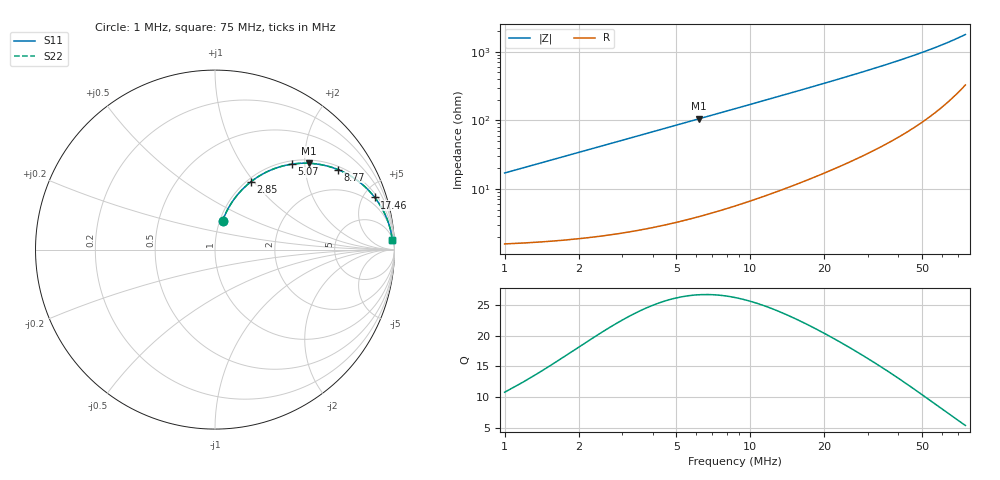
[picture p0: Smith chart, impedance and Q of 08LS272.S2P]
! Coilcraft 0805LS-272 Chip Inductor
! 18 September 2002
# MHZ S MA R 50
!Freq  MagS11  AngS11  MagS21  AngS21  MagS12  AngS12  MagS22  AngS22
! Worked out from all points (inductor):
!   401 points, 1 MHz to 75 MHz, reference 50 ohm
!   read as one part in series: L = 2.7 uH near 1.37 MHz
!   highest Q = 26.7 at 6.18 MHz (marker M1), where L = 2.7 uH
!   S11 on the Smith chart (normalised r, x): 1 MHz: 1.03, +0.34; 2.85 MHz: 1.04, +0.97; 5.07 MHz: 1.07, +1.72; 8.77 MHz: 1.11, +2.99; 17.46 MHz: 1.28, +6.02; 75 MHz: 8, +35
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1  0.1654 75.2  0.971 -9.5  0.971 -9.5  0.1654 75.2
1.185  0.1947 74.2  0.9653 -11.2  0.9653 -11.2  0.1947 74.2
1.555  0.2515 71.7  0.9515 -14.5  0.9515 -14.5  0.2515 71.7
1.925  0.3058 69.0  0.935 -17.8  0.935 -17.8  0.3058 69.0
2.295  0.3572 66.2  0.9161 -20.9  0.9161 -20.9  0.3572 66.2
2.85  0.4281 62.1  0.8845 -25.3  0.8845 -25.3  0.4281 62.1
3.775  0.5301 55.7  0.8266 -32.0  0.8266 -32.0  0.5301 55.7
4.33  0.5817 52.2  0.7908 -35.5  0.7908 -35.5  0.5817 52.2
5.07  0.6407 48.0  0.7437 -39.8  0.7437 -39.8  0.6407 48.0
6.18  0.7112 42.6  0.6769 -45.3  0.6769 -45.3  0.7112 42.6
7.475  0.7722 37.3  0.6071 -50.5  0.6071 -50.5  0.7722 37.3
8.77  0.8167 33.1  0.5467 -54.7  0.5467 -54.7  0.8167 33.1
10.805  0.8648 27.9  0.4689 -59.8  0.4689 -59.8  0.8648 27.9
13.395  0.9029 23.2  0.3936 -64.4  0.3936 -64.4  0.9029 23.2
17.465  0.9362 18.1  0.3109 -69.3  0.3109 -69.3  0.9362 18.1
21.165  0.9529 15.0  0.2592 -72.1  0.2592 -72.1  0.9529 15.0
25.79  0.9653 12.3  0.2129 -74.5  0.2129 -74.5  0.9653 12.3
31.525  0.9741 9.9  0.1726 -76.4  0.1726 -76.4  0.9741 9.9
38  0.9799 8.1  0.1405 -77.8  0.1405 -77.8  0.9799 8.1
50.395  0.9854 5.7  0.09993 -78.7  0.09993 -78.7  0.9854 5.7
62.79  0.9876 4.2  0.07376 -78.2  0.07376 -78.2  0.9876 4.2
75  0.9884 3.1  0.05537 -76.3  0.05537 -76.3  0.9884 3.1
